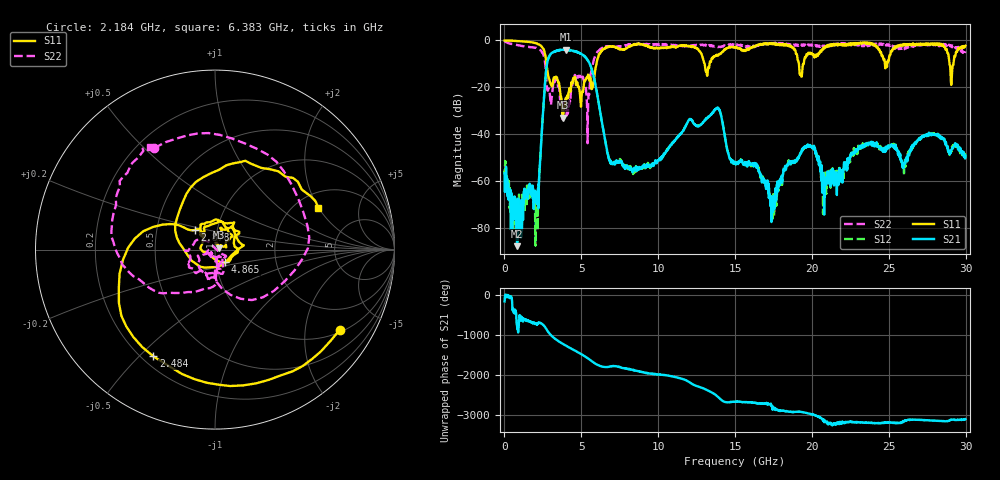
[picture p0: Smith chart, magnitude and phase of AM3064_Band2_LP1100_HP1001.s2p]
# Hz S DB R 50.0
!freq dBS11 angS11 dBS21 angS21 dBS12 angS12 dBS22 angS22
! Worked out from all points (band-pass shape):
!   1600 points, 10 MHz to 29.98 GHz, reference 50 ohm
!   highest |S21| = -3.92 dB at 4.002 GHz (marker M1); lowest = -87.9 dB at 816 MHz (marker M2)
!   |S21| within 3 dB of the highest: 2.907 GHz to 5.209 GHz (2.302 GHz wide, 56.7 % of centre)
!   lowest |S11| = -33.0 dB at 3.796 GHz (marker M3), VSWR 1.05, Z = 52 + j1.15 ohm
!   |S11| at or under -10 dB: 2.731 GHz to 5.984 GHz (3.253 GHz wide, 74.7 % of centre); 13.02 GHz to 13.34 GHz (324 MHz wide, 2.46 % of centre); 19.15 GHz to 19.47 GHz (315.4 MHz wide, 1.63 % of centre)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
!   |S22| runs from -43.9 to -0.3 dB; largest |S21 - S12| = 0.018
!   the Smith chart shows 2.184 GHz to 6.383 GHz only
!   S11 on the Smith chart (normalised r, x): 2.184 GHz: 1.09, -3.06; 2.484 GHz: 0.24, -0.55; 2.878 GHz: 0.78, +0.17; 4.865 GHz: 1.11, -0.16; 6.383 GHz: 2.62, +1.99
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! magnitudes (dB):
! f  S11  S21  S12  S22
! 10 MHz  -0.1  -56.9  -55.0  -0.3
! 816 MHz  -0.3  -87.9  -75.4  -2.0
! 2.184 GHz  -1.7  -63.3  -65.2  -3.6
! 2.484 GHz  -3.3  -33.3  -33.3  -5.5
! 2.878 GHz  -16.1  -7.3  -7.3  -20.6
! 3.796 GHz  -33.0  -4.0  -3.9  -30.2
! 4.002 GHz  -24.5  -3.9  -4.1  -28.4
! 4.865 GHz  -20.8  -5.3  -5.3  -15.4
! 5.015 GHz  -24.0  -5.9  -5.8  -16.9
! 5.408 GHz  -15.3  -8.3  -8.4  -43.9
! 6.383 GHz  -4.1  -36.6  -36.6  -3.4
! 6.983 GHz  -2.6  -52.8  -52.7  -2.7
! 10 GHz  -3.4  -51.4  -51.3  -1.8
! 13.82 GHz  -6.2  -28.8  -29.0  -2.7
! 15 GHz  -2.9  -52.9  -52.4  -1.9
! 17.46 GHz  -1.3  -70.0  -72.8  -1.4
! 19.99 GHz  -5.5  -45.8  -45.3  -1.8
! 20.82 GHz  -3.0  -62.4  -63.0  -2.3
! 25 GHz  -8.6  -45.8  -45.5  -1.8
! 28.28 GHz  -1.3  -41.4  -41.0  -2.6
! 29.08 GHz  -17.8  -46.8  -47.4  -2.6
! 29.98 GHz  -2.3  -49.2  -50.4  -4.7
